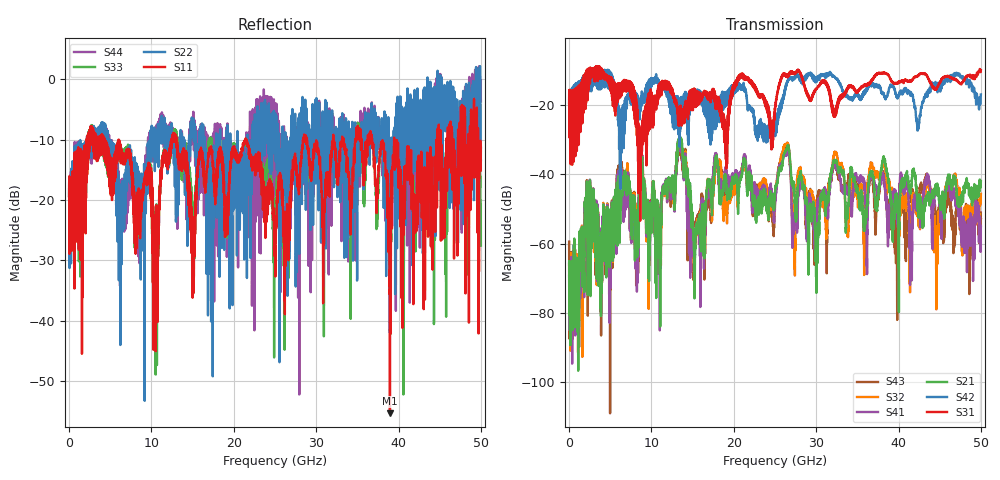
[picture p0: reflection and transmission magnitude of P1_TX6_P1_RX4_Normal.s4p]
!Keysight Technologies,N5225B,MY57041031,A.13.20.10
!Date: Friday, May 31, 2019 11:19:21
!Correction: S11(Full 4 Port(1,2,3,4))
!S12(Full 4 Port(1,2,3,4))
!S13(Full 4 Port(1,2,3,4))
!S14(Full 4 Port(1,2,3,4))
!S21(Full 4 Port(1,2,3,4))
!S22(Full 4 Port(1,2,3,4))
!S23(Full 4 Port(1,2,3,4))
!S24(Full 4 Port(1,2,3,4))
!S31(Full 4 Port(1,2,3,4))
!S32(Full 4 Port(1,2,3,4))
!S33(Full 4 Port(1,2,3,4))
!S34(Full 4 Port(1,2,3,4))
!S41(Full 4 Port(1,2,3,4))
!S42(Full 4 Port(1,2,3,4))
!S43(Full 4 Port(1,2,3,4))
!S44(Full 4 Port(1,2,3,4))
!S4P File: Measurements: <S11,S12,S13,S14>,
!<S21,S22,S23,S24>,
!<S31,S32,S33,S34>,
!<S41,S42,S43,S44>:
# Hz S  dB  R 50.0
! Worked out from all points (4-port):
!   5000 points, 10 MHz to 50 GHz, reference 50 ohm
!   strongest paths, dB at 10 MHz, 12.51 GHz, 25.01 GHz, 37.51 GHz, 50 GHz:
!     S31: -19.4, -15.5, -21.6, -10.8, -9.9
!     S42: -19.4, -19.3, -26.0, -14.8, -16.9
!     S21: -65.5, -42.0, -45.2, -46.7, -41.9
!     S41: -69.2, -42.5, -48.5, -45.2, -55.2
!     S32: -66.2, -43.5, -45.7, -40.6, -45.7
!     S43: -59.5, -44.0, -47.9, -46.2, -52.9
!   lowest |S11| = -55.3 dB at 38.96 GHz (marker M1), VSWR 1.00, Z = 50.1 + j0.151 ohm
!   |S11| at or under -10 dB: 4.286 GHz to 12.47 GHz (8.179 GHz wide, 97.6 % of centre); 13.02 GHz to 21.43 GHz (8.403 GHz wide, 48.8 % of centre); 21.46 GHz to 28.42 GHz (6.96 GHz wide, 27.9 % of centre)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
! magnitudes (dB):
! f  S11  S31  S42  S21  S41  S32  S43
! 10 MHz  -19.3  -19.4  -19.4  -65.5  -69.2  -66.2  -59.5
! 13.42 GHz  -13.4  -24.7  -32.1  -29.5  -30.4  -30.6  -31.8
! 15.32 GHz  -22.7  -17.5  -16.3  -60.5  -59.5  -56.7  -55.2
! 17.81 GHz  -17.9  -17.6  -26.9  -35.4  -34.5  -37.9  -37.1
! 30.11 GHz  -10.4  -15.1  -12.1  -61.6  -51.0  -52.1  -48.5
! 38.96 GHz  -55.3  -12.3  -14.5  -44.8  -49.6  -43.8  -53.6
! 50 GHz  -11.3  -9.9  -16.9  -41.9  -55.2  -45.7  -52.9
